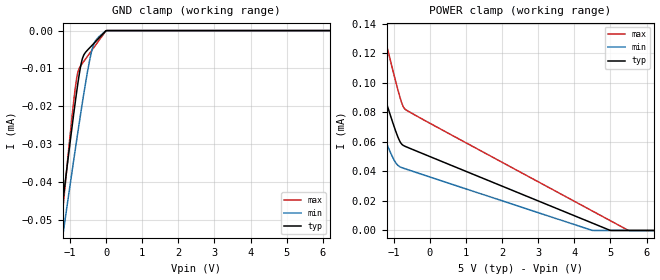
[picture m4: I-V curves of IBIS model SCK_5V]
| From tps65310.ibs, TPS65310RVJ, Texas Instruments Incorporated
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[Model]   SCK_5V
Model_type   Input
Vinl = .8
Vinh = 2.
|   typ   min   max
C_comp   0.01p   0.01p   0.01p
[Voltage Range]   5   4.5   5.5
[Temperature Range]   27   175   -40
[Power Clamp Reference]   5   4.5   5.5
[GND Clamp Reference]   -0   -0   -0
[GND Clamp]
|   Voltage   I(typ)   I(min)   I(max)
-5V       -355.8uA   -316.3uA   -439.7uA
-1.46V    -66.04uA   -71.8uA    -73.56uA
-1.25V    -49.29uA   -57.63uA   -52.4uA
-1.07V    -35.16uA   -45.62uA   -34.65uA
-875mV    -20.43uA   -32.82uA   -16.84uA
-785mV    -14.16uA   -27.04uA   -11.13uA
-650mV    -7.221uA   -18.63uA   -8.578uA
-515mV    -5.161uA   -10.84uA   -6.793uA
-395mV    -3.952uA   -5.266uA   -5.21uA
-290mV    -2.901uA   -2.635uA   -3.825uA
-5mV      -48.51nA   -38.61nA   -64.49nA
9.985V    0A         0A         0A
[POWER Clamp]
|   Voltage   I(typ)   I(min)   I(max)
-5V       395.6uA    318.2uA    517.6uA
-2.36V    179.3uA    136uA      244.3uA
-1.985V   148.8uA    110.5uA    205.7uA
-1.745V   129.4uA    94.4uA     181.1uA
-1.445V   105.4uA    74.6uA     150.5uA
-1.25V    90.02uA    62.19uA    130.8uA
-965mV    68.59uA    46.6uA     102.7uA
-770mV    58.22uA    42.5uA     85.77uA
-410mV    54.17uA    39.53uA    78.13uA
4.495V    5.053uA    38.62nA    13.26uA
5.485V    0A         0A         196.4nA
9.985V    0A         0A         0A
